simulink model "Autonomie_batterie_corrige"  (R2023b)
settings: Solver=VariableStepAuto  StartTime=0.0  StopTime=15000  RelTol=1e-3
libraries: fl_lib x9, nesl_utility x4, fl_ps_legacy_lib x2, batteryecm_lib x1

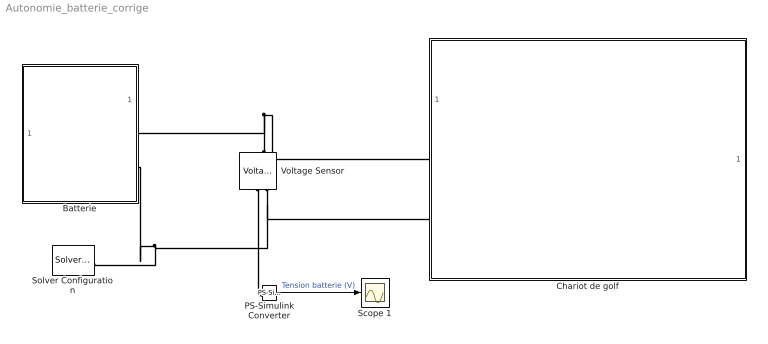
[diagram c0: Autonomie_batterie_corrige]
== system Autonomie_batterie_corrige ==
  Batterie : Subsystem  mask{U=14.8, Rbat=0.1, Q=16, Pd=80}
      mask prompts: U "Tension Batterie en V"; Rbat "Résistance interne en Ohm"; Q "Capacité en Ah"; Pd "Profondeur de décharge en %"
  Chariot de golf : Subsystem
  PS-Simulink Converter : nesl_utility/PS-Simulink Converter  PhysicalDomain=network_engine_domain  SubClassName=ps_output  LeftPortType=input  RightPortType=output  PseudoPeriodic=off  Frequencies=[]  VectorFormat=inherit  Unit=V  AffineConversion=off
  Scope 1 : Scope
  Solver Configuration : nesl_utility/Solver Configuration  PhysicalDomain=network_engine_domain  SubClassName=solver  LeftPortType=input  RightPortType=generic  Tones=[]  Harmonics=[]  SimulateNoise=off  Profile=off  UseLocalSampling=off  EnableSwitchedLinearOptims=on  FrequencyDomain=off  UseCCode=off  RelTol=0.001  AbsTol=0.001  MinStep=1e-09  ToWorkspace=off  RevertToSquareIcSolve=off  NumHomotopyIterations=100  PhasorMode=off  PhasorModeNumHarmonics=1  ConsistencySolver=NEWTON_XTOL_AFTER_FTOL  IndexReductionMethod=DerivativeReplacement  DoDC=off  ResidualTolerance=1e-09  ConsistencyTolSource=GLOBAL  ConsistencyAbsTol=0.001  ConsistencyRelTol=0.001  ConsistencyTolFactor=0.001  UseLocalSolver=off  LocalSolverChoice=NE_BACKWARD_EULER_ADVANCER  ResolveIndetEquations=on  FunctionEvalNumThread=1  LocalSolverSampleTime=0.001  DoFixedCost=off  MaxNonlinIter=3  MaxModeIter=2  ComputeImpulses=off  ImpulseIterations=2  LinearAlgebra=auto  LinearAlgebraNumThread=0  EquationFormulation=NE_TIME_EF  DelaysMemoryBudget=1024  AutomaticFiltering=on  FilteringTimeConstant=0.001  PartitionStorageMethod=AS_NEEDED  PartitionMemoryBudget=1024  PartitionMethod=ROBUST  MultibodyUseLocalSolver=off  MultibodyLocalSolverChoice=ODE1  MultibodyLocalSolverSampleTime=0.001
  Voltage Sensor : fl_lib/Electrical/Electrical Sensors/Voltage Sensor
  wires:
  PS-Simulink Converter/1 -> Scope 1/1  "Tension batterie (V)"
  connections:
  Voltage Sensor/RConn1 -- PS-Simulink Converter/LConn1
  Voltage Sensor/LConn1 -- Batterie/RConn1 -- Chariot de golf/LConn1
  Voltage Sensor/RConn2 -- Batterie/RConn2 -- Solver Configuration/RConn1 -- Chariot de golf/LConn2

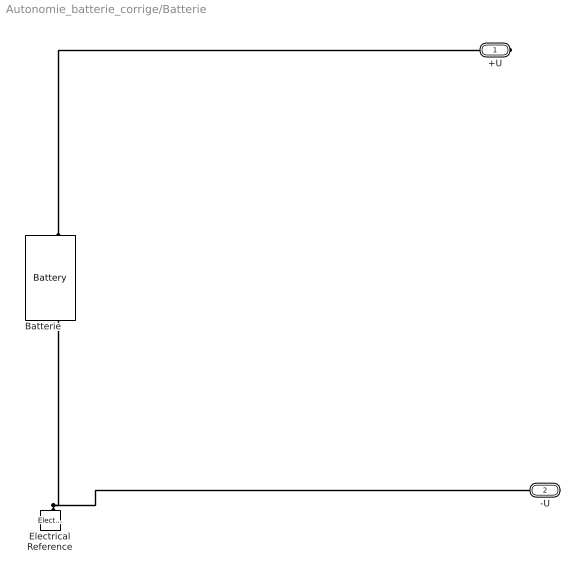
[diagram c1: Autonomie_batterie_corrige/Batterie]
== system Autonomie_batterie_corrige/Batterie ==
  Batterie : batteryecm_lib/Battery  Vnom=U V  prm_dir=simscape.enum.battery.prm_dir.disabled  R1_dis=2 Ohm  R1_ch=2 Ohm  R1=Rbat Ohm  prm_AH=2  AH=Q hr*A  V1=.8*U V  AH1=Pd*Q/100 hr*A  prm_R2=1  R2=2000 Ohm  Tmeas=298.15 K  charge_measurement_port=simscape.enum.battery.enable.no  prm_dyn=simscape.enum.battery.prm_dyn.off  Rp1=0.005 Ohm  tau1=30 s  Rp2=0.005 Ohm  tau2=30 s  Rp3=0.005 Ohm  tau3=30 s  Rp4=0.005 Ohm  tau4=30 s  Rp5=0.005 Ohm  tau5=30 s  prm_fade=simscape.enum.battery.prm_fade.disabled  N_fade=100  AH_fade=45 A*hr  R1_fade=2.02 Ohm  R1_ch_fade=2.02 Ohm  V1_fade=10.35 V  prm_age=simscape.enum.battery.prm_age.disabled  prm_age_OCV=simscape.enum.battery.prm_age_OCV.OCV  OCV_age=0.9  SOC_age=60  Tmeas_age=298.15 K  delta_time_age_vec=[0] d  temperature_age_vec=[273] K  OCV_scaling_age=2.2134e6  OCV_offset_age=1.632e6  temp_exp_age=0.515833569 V  t_exp_age=0.75  Vnom_T2=12 V  R1_T2=2.2 Ohm  R1_T2_dis=2.2 Ohm  R1_T2_ch=2.2 Ohm  V1_T2=11.4 V  R2_T2=2200 Ohm  Rp1_T2=0.005 Ohm  tau1_T2=30 s  Rp2_T2=0.005 Ohm  tau2_T2=30 s  Rp3_T2=0.005 Ohm  tau3_T2=30 s  Rp4_T2=0.005 Ohm  tau4_T2=30 s  Rp5_T2=0.005 Ohm  tau5_T2=30 s  Tmeas2=273.15 K  thermal_port=simscape.enum.thermaleffects.omit  thermal_mass=30000 J/K  i_specify=off  i_priority=None  i=0 A  i_nominal_specify=off  i_nominal_unit=A  i_nominal_value=1  v_specify=off  v_priority=None  v=0 V  v_nominal_specify=off  v_nominal_unit=V  v_nominal_value=1  charge_specify=on  charge_priority=High  charge=Q hr*A  charge_nominal_specify=off  charge_nominal_unit=A*hr  charge_nominal_value=1  num_cycles_specify=off  num_cycles_priority=High  num_cycles=0  num_cycles_nominal_specify=off  num_cycles_nominal_unit=1  num_cycles_nominal_value=1  temperature_specify=off  temperature_priority=High  temperature=298.15 K  temperature_nominal_specify=off  temperature_nominal_unit=K  temperature_nominal_value=1
  Electrical Reference : fl_lib/Electrical/Electrical Elements/Electrical Reference
  +U : PMIOPort  Side=Right
  -U : PMIOPort  Port=2  Side=Right
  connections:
  Electrical Reference/LConn1 -- -U/RConn1 -- Batterie/RConn1
  Batterie/LConn1 -- +U/RConn1

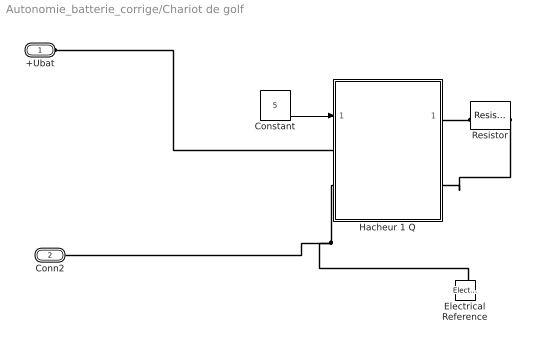
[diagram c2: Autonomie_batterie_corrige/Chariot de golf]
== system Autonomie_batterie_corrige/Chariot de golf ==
  Constant : Constant  Value=5
  Electrical Reference : fl_lib/Electrical/Electrical Elements/Electrical Reference
  Hacheur 1 Q : Subsystem
      mask init:
      | F_decou=490;
  Resistor : fl_lib/Electrical/Electrical Elements/Resistor  R=3 Ohm  i_specify=off  i_priority=None  i=0 A  i_nominal_specify=off  i_nominal_unit=A  i_nominal_value=1  v_specify=off  v_priority=None  v=0 V  v_nominal_specify=off  v_nominal_unit=V  v_nominal_value=1
  +Ubat : PMIOPort  Side=Left
  Conn2 : PMIOPort  Port=2  Side=Left
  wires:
  Constant/1 -> Hacheur 1 Q/1(Consigne)
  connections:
  Hacheur 1 Q/RConn1 -- Resistor/LConn1
  Hacheur 1 Q/LConn2 -- Electrical Reference/LConn1 -- Conn2/RConn1
  Hacheur 1 Q/LConn1 -- +Ubat/RConn1
  Resistor/RConn1 -- Hacheur 1 Q/RConn2

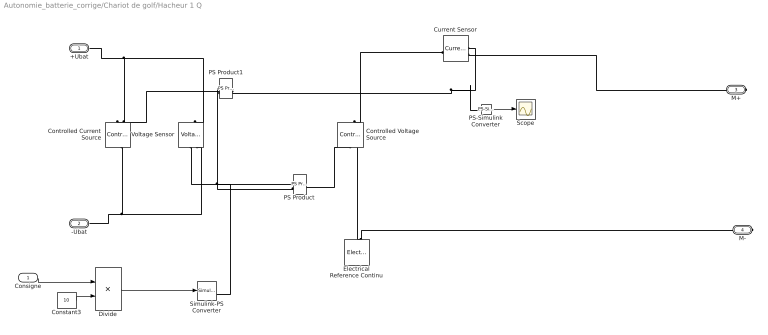
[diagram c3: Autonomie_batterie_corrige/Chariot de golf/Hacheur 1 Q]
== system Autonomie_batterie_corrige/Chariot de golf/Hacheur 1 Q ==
  Consigne : Inport
  Constant3 : Constant  Value=10
  Controlled Current Source : fl_lib/Electrical/Electrical Sources/Controlled Current Source
  Controlled Voltage Source : fl_lib/Electrical/Electrical Sources/Controlled Voltage Source
  Current Sensor : fl_lib/Electrical/Electrical Sensors/Current Sensor
  Divide : Product  Inputs=*/
  Electrical Reference Continu : fl_lib/Electrical/Electrical Elements/Electrical Reference
  PS Product : fl_ps_legacy_lib/Legacy Physical Signals/Functions/PS Product
  PS Product1 : fl_ps_legacy_lib/Legacy Physical Signals/Functions/PS Product
  PS-Simulink Converter : nesl_utility/PS-Simulink Converter  PhysicalDomain=network_engine_domain  SubClassName=ps_output  LeftPortType=input  RightPortType=output  PseudoPeriodic=off  Frequencies=[]  VectorFormat=inherit  Unit=inherit  AffineConversion=off
  Scope : Scope
  Simulink-PS Converter : nesl_utility/Simulink-PS Converter  PhysicalDomain=network_engine_domain  SubClassName=ps_input  LeftPortType=input  RightPortType=output  PseudoPeriodic=off  Frequencies=[]  NoiseDistribution=none  NoiseParameters=[]  Unit=1  AffineConversion=off  FilteringAndDerivatives=zero  SimscapeFilterOrder=1  InputFilterTimeConstant=0.001  UdotUserProvided=1
  Voltage Sensor : fl_lib/Electrical/Electrical Sensors/Voltage Sensor
  +Ubat : PMIOPort  Side=Left
  -Ubat : PMIOPort  Port=2  Side=Left
  M+ : PMIOPort  Port=3  Side=Right
  M- : PMIOPort  Port=4  Side=Right
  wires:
  Consigne/1 -> Divide/1
  Constant3/1 -> Divide/2
  Divide/1 -> Simulink-PS Converter/1
  PS-Simulink Converter/1 -> Scope/1
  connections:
  Controlled Current Source/LConn1 -- -Ubat/RConn1 -- Voltage Sensor/RConn2
  Controlled Current Source/RConn2 -- +Ubat/RConn1 -- Voltage Sensor/LConn1
  PS Product1/LConn1 -- PS Product/LConn2 -- Simulink-PS Converter/RConn1
  Current Sensor/LConn1 -- Controlled Voltage Source/LConn1
  Voltage Sensor/RConn1 -- PS Product/LConn1
  PS Product1/RConn1 -- Controlled Current Source/RConn1
  PS Product/RConn1 -- Controlled Voltage Source/RConn1
  Current Sensor/RConn1 -- PS-Simulink Converter/LConn1 -- PS Product1/LConn2
  Electrical Reference Continu/LConn1 -- Controlled Voltage Source/RConn2 -- M-/RConn1
  Current Sensor/RConn2 -- M+/RConn1
